(* Logix 5000 AddOnInstructionDefinition export Banner_Q5X_Jam_Param_v4; software revision 33.00; part 2 of 3 *)
(* tags used below, declared in another part *)
   Q5X : Banner_Q5X_Jam_v4;
   Port_Data : Banner_IOL_Port_v4;
   Port : DINT;
   Local_Control : DINT;
   Command_Being_Processed : BOOL;
   Update_Archive : BOOL;
   Index_Write_Inprocess : INT;
   Index_Write_Control : INT;
   Inprocess_Index : DINT;
(* Banner_Q5X_Jam_Param_v4, continued *)

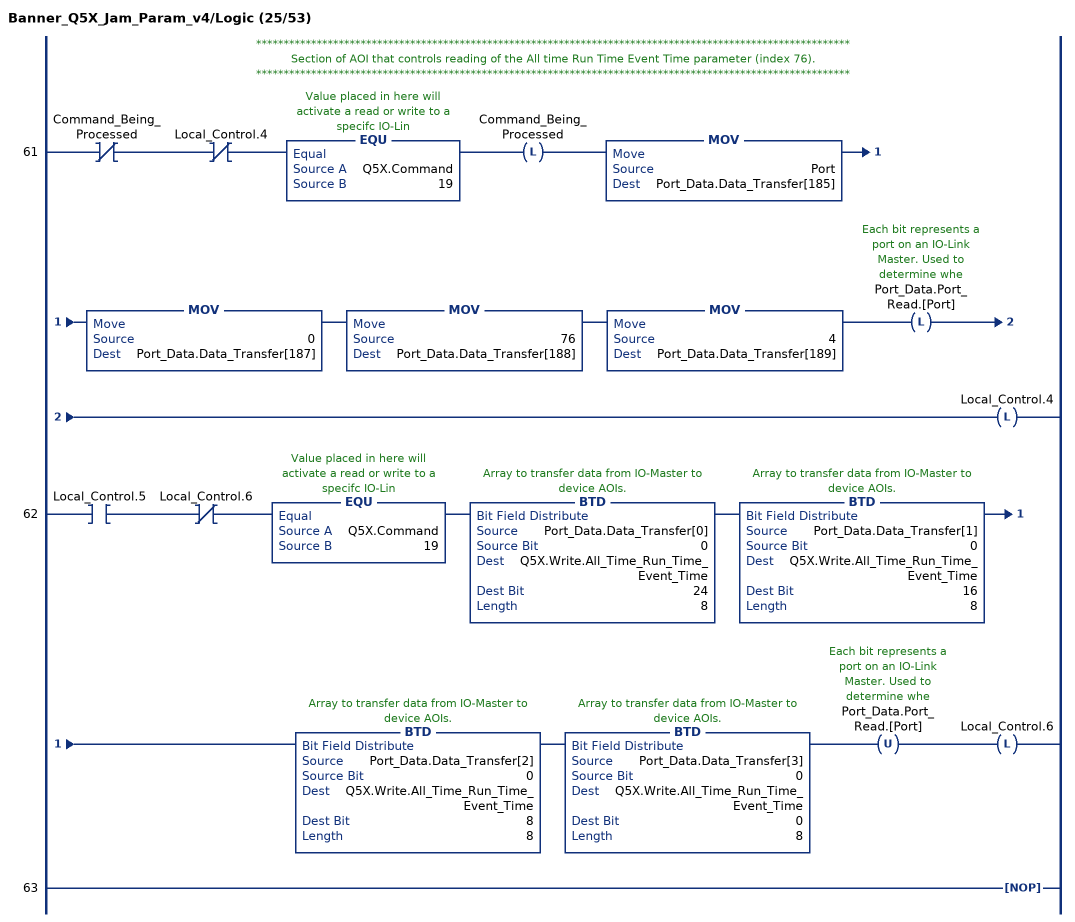
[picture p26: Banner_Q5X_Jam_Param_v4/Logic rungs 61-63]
   // ************************************************************************************************************
   // Section of AOI that controls reading of the All time Run Time Event Time parameter (index 76).
   // ************************************************************************************************************
   61: XIO(Command_Being_Processed)XIO(Local_Control.4)EQU(Q5X.Command,19)OTL(Command_Being_Processed)MOV(Port,Port_Data.Data_Transfer[185])MOV(0,Port_Data.Data_Transfer[187])MOV(76,Port_Data.Data_Transfer[188])MOV(4,Port_Data.Data_Transfer[189])OTL(Port_Data.Port_Read.[Port])OTL(Local_Control.4);
   62: XIC(Local_Control.5)XIO(Local_Control.6)EQU(Q5X.Command,19)BTD(Port_Data.Data_Transfer[0],0,Q5X.Write.All_Time_Run_Time_Event_Time,24,8)BTD(Port_Data.Data_Transfer[1],0,Q5X.Write.All_Time_Run_Time_Event_Time,16,8)BTD(Port_Data.Data_Transfer[2],0,Q5X.Write.All_Time_Run_Time_Event_Time,8,8)BTD(Port_Data.Data_Transfer[3],0,Q5X.Write.All_Time_Run_Time_Event_Time,0,8)OTU(Port_Data.Port_Read.[Port])OTL(Local_Control.6);
   63: NOP();
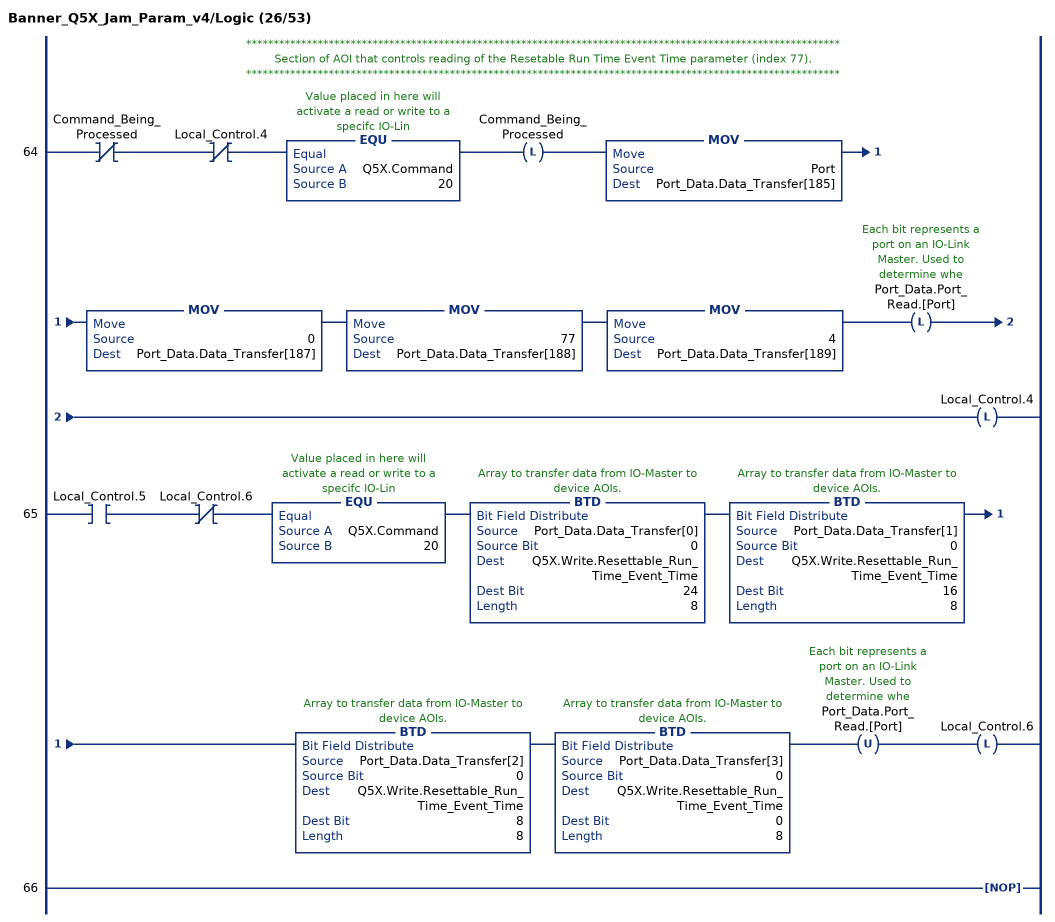
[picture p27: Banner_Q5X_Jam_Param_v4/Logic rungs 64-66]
   // ************************************************************************************************************
   // Section of AOI that controls reading of the Resetable Run Time Event Time parameter (index 77).
   // ************************************************************************************************************
   64: XIO(Command_Being_Processed)XIO(Local_Control.4)EQU(Q5X.Command,20)OTL(Command_Being_Processed)MOV(Port,Port_Data.Data_Transfer[185])MOV(0,Port_Data.Data_Transfer[187])MOV(77,Port_Data.Data_Transfer[188])MOV(4,Port_Data.Data_Transfer[189])OTL(Port_Data.Port_Read.[Port])OTL(Local_Control.4);
   65: XIC(Local_Control.5)XIO(Local_Control.6)EQU(Q5X.Command,20)BTD(Port_Data.Data_Transfer[0],0,Q5X.Write.Resettable_Run_Time_Event_Time,24,8)BTD(Port_Data.Data_Transfer[1],0,Q5X.Write.Resettable_Run_Time_Event_Time,16,8)BTD(Port_Data.Data_Transfer[2],0,Q5X.Write.Resettable_Run_Time_Event_Time,8,8)BTD(Port_Data.Data_Transfer[3],0,Q5X.Write.Resettable_Run_Time_Event_Time,0,8)OTU(Port_Data.Port_Read.[Port])OTL(Local_Control.6);
   66: NOP();
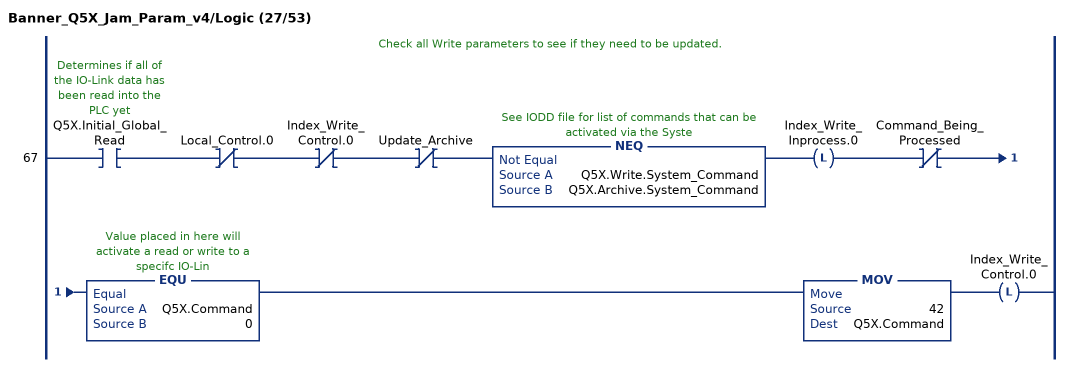
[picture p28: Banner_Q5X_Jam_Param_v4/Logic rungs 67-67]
   // Check all Write parameters to see if they need to be updated.
   67: XIC(Q5X.Initial_Global_Read)XIO(Local_Control.0)XIO(Index_Write_Control.0)XIO(Update_Archive)NEQ(Q5X.Write.System_Command,Q5X.Archive.System_Command)OTL(Index_Write_Inprocess.0)XIO(Command_Being_Processed)EQU(Q5X.Command,0)MOV(42,Q5X.Command)OTL(Index_Write_Control.0);
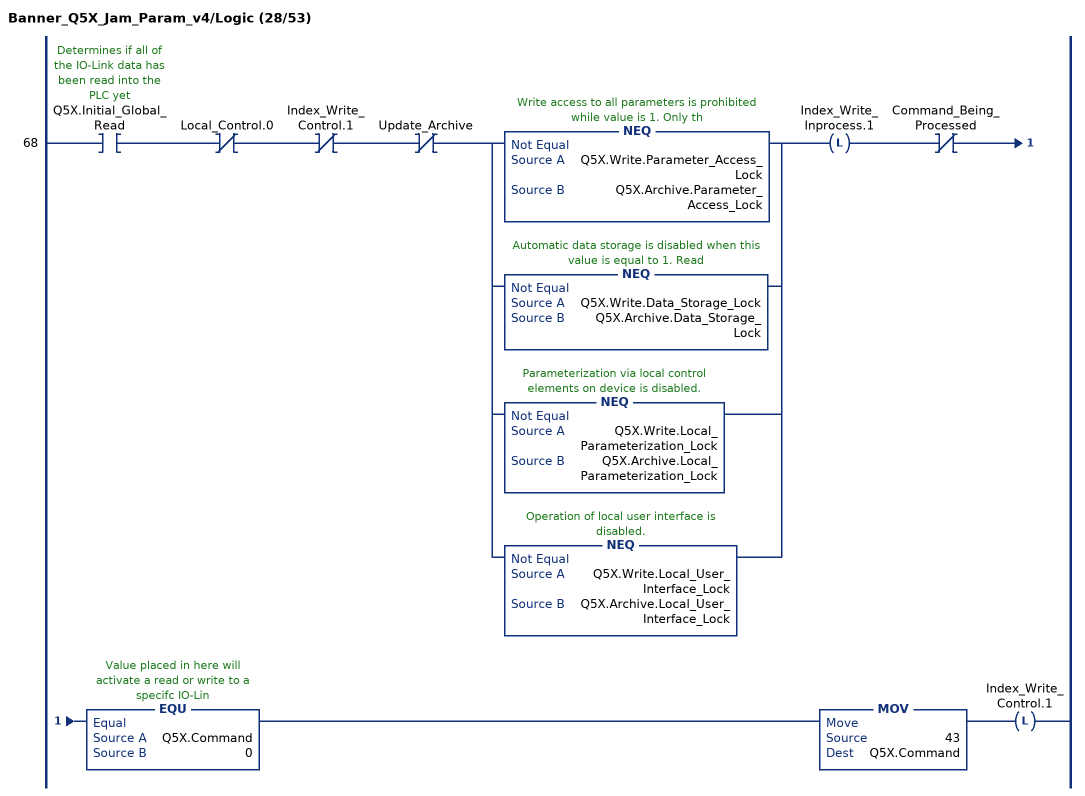
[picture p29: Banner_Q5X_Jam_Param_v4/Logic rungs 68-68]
   68: XIC(Q5X.Initial_Global_Read)XIO(Local_Control.0)XIO(Index_Write_Control.1)XIO(Update_Archive)[NEQ(Q5X.Write.Parameter_Access_Lock,Q5X.Archive.Parameter_Access_Lock) ,NEQ(Q5X.Write.Data_Storage_Lock,Q5X.Archive.Data_Storage_Lock) ,NEQ(Q5X.Write.Local_Parameterization_Lock,Q5X.Archive.Local_Parameterization_Lock) ,NEQ(Q5X.Write.Local_User_Interface_Lock,Q5X.Archive.Local_User_Interface_Lock) ]OTL(Index_Write_Inprocess.1)XIO(Command_Being_Processed)EQU(Q5X.Command,0)MOV(43,Q5X.Command)OTL(Index_Write_Control.1);
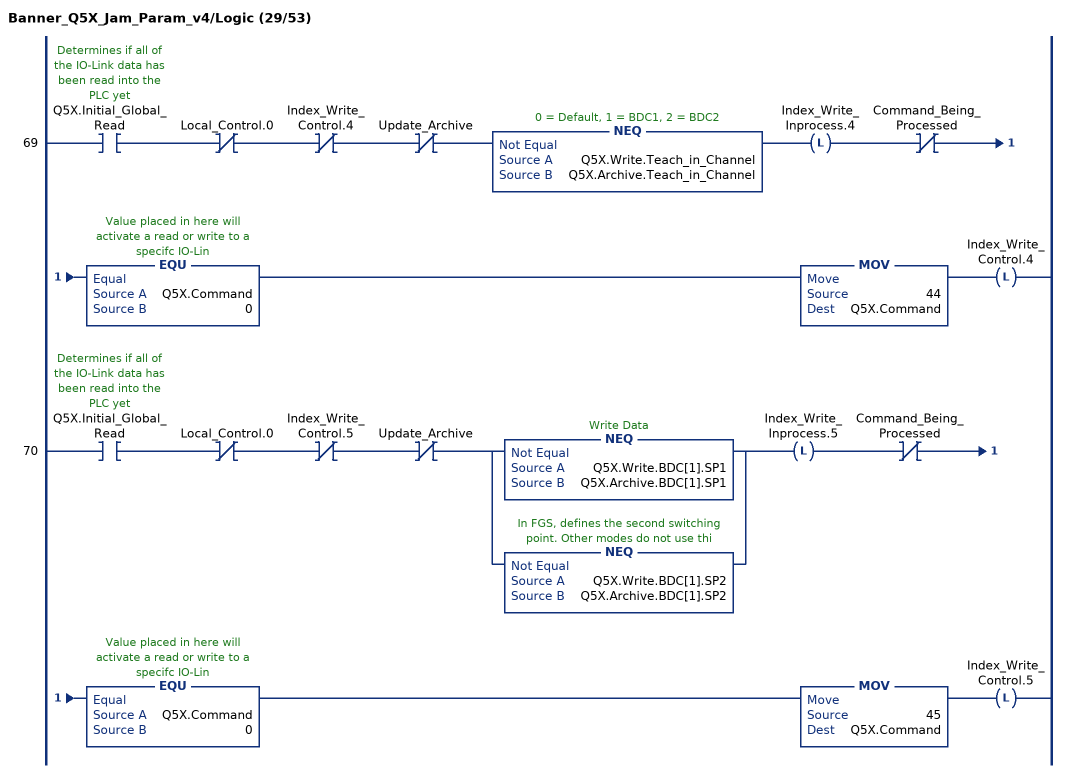
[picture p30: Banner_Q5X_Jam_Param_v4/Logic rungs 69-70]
   69: XIC(Q5X.Initial_Global_Read)XIO(Local_Control.0)XIO(Index_Write_Control.4)XIO(Update_Archive)NEQ(Q5X.Write.Teach_in_Channel,Q5X.Archive.Teach_in_Channel)OTL(Index_Write_Inprocess.4)XIO(Command_Being_Processed)EQU(Q5X.Command,0)MOV(44,Q5X.Command)OTL(Index_Write_Control.4);
   70: XIC(Q5X.Initial_Global_Read)XIO(Local_Control.0)XIO(Index_Write_Control.5)XIO(Update_Archive)[NEQ(Q5X.Write.BDC[1].SP1,Q5X.Archive.BDC[1].SP1) ,NEQ(Q5X.Write.BDC[1].SP2,Q5X.Archive.BDC[1].SP2) ]OTL(Index_Write_Inprocess.5)XIO(Command_Being_Processed)EQU(Q5X.Command,0)MOV(45,Q5X.Command)OTL(Index_Write_Control.5);
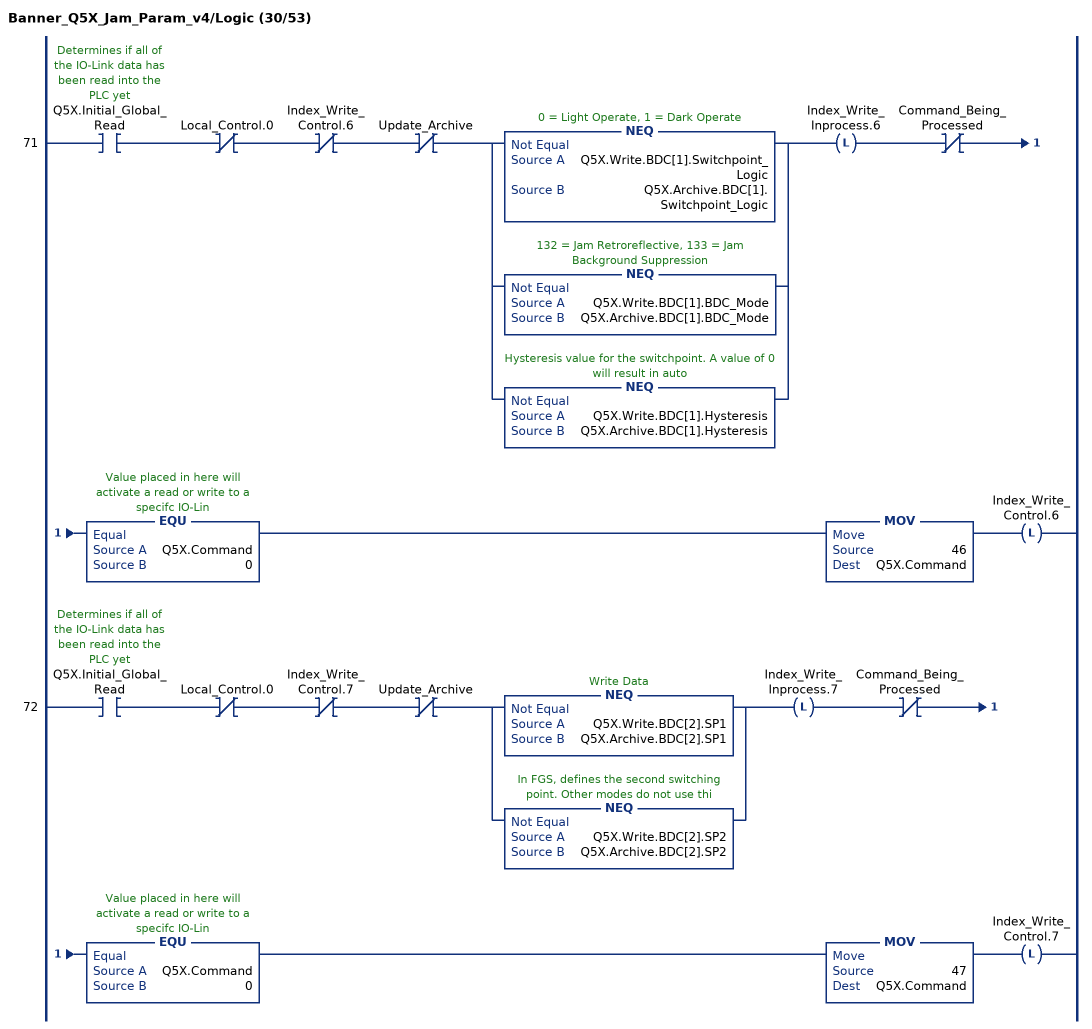
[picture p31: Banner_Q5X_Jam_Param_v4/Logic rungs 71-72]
   71: XIC(Q5X.Initial_Global_Read)XIO(Local_Control.0)XIO(Index_Write_Control.6)XIO(Update_Archive)[NEQ(Q5X.Write.BDC[1].Switchpoint_Logic,Q5X.Archive.BDC[1].Switchpoint_Logic) ,NEQ(Q5X.Write.BDC[1].BDC_Mode,Q5X.Archive.BDC[1].BDC_Mode) ,NEQ(Q5X.Write.BDC[1].Hysteresis,Q5X.Archive.BDC[1].Hysteresis) ]OTL(Index_Write_Inprocess.6)XIO(Command_Being_Processed)EQU(Q5X.Command,0)MOV(46,Q5X.Command)OTL(Index_Write_Control.6);
   72: XIC(Q5X.Initial_Global_Read)XIO(Local_Control.0)XIO(Index_Write_Control.7)XIO(Update_Archive)[NEQ(Q5X.Write.BDC[2].SP1,Q5X.Archive.BDC[2].SP1) ,NEQ(Q5X.Write.BDC[2].SP2,Q5X.Archive.BDC[2].SP2) ]OTL(Index_Write_Inprocess.7)XIO(Command_Being_Processed)EQU(Q5X.Command,0)MOV(47,Q5X.Command)OTL(Index_Write_Control.7);
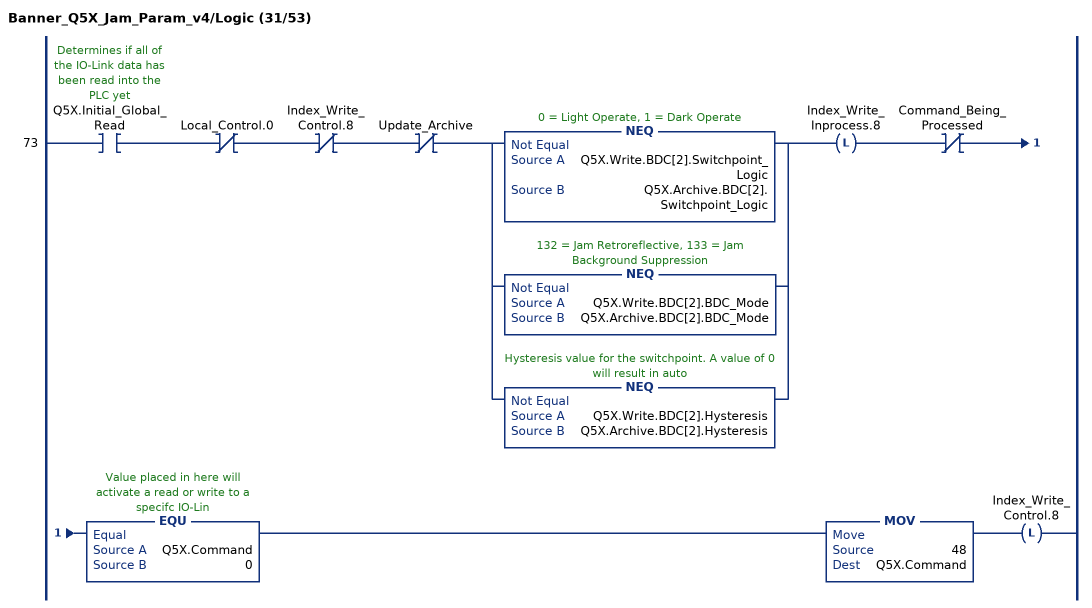
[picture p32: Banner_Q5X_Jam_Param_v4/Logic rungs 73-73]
   73: XIC(Q5X.Initial_Global_Read)XIO(Local_Control.0)XIO(Index_Write_Control.8)XIO(Update_Archive)[NEQ(Q5X.Write.BDC[2].Switchpoint_Logic,Q5X.Archive.BDC[2].Switchpoint_Logic) ,NEQ(Q5X.Write.BDC[2].BDC_Mode,Q5X.Archive.BDC[2].BDC_Mode) ,NEQ(Q5X.Write.BDC[2].Hysteresis,Q5X.Archive.BDC[2].Hysteresis) ]OTL(Index_Write_Inprocess.8)XIO(Command_Being_Processed)EQU(Q5X.Command,0)MOV(48,Q5X.Command)OTL(Index_Write_Control.8);
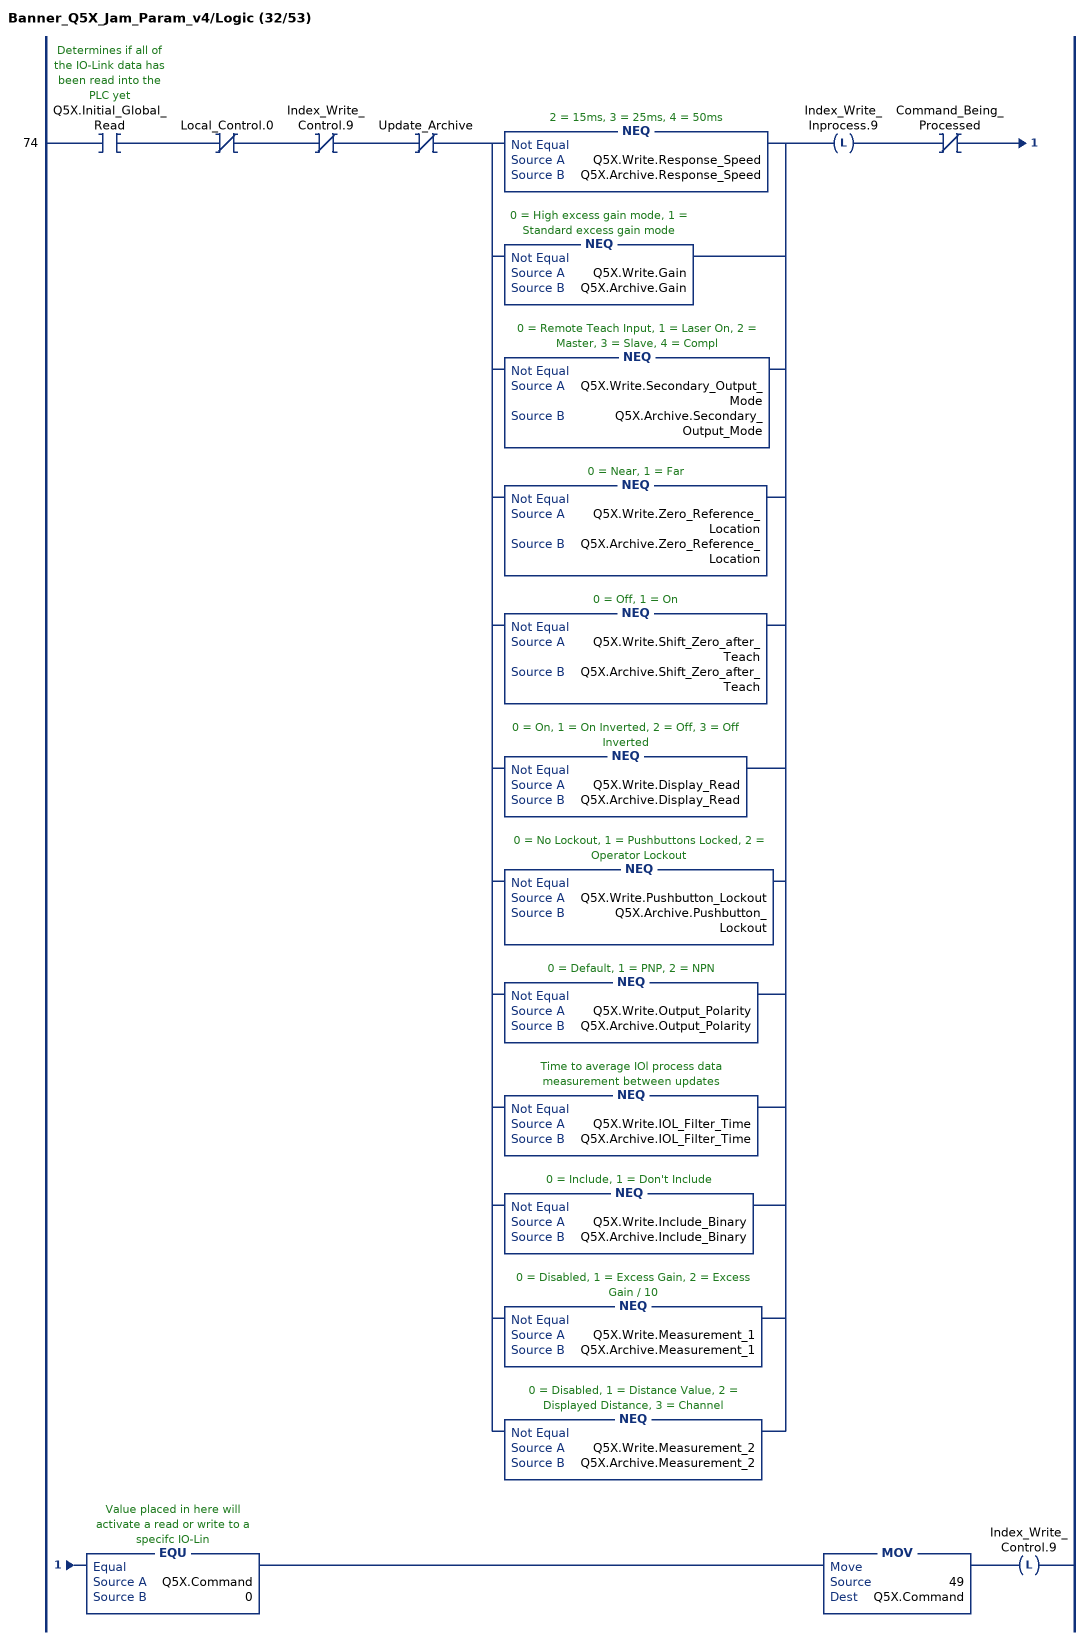
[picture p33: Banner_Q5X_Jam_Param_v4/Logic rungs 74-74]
   74: XIC(Q5X.Initial_Global_Read)XIO(Local_Control.0)XIO(Index_Write_Control.9)XIO(Update_Archive)[NEQ(Q5X.Write.Response_Speed,Q5X.Archive.Response_Speed) ,NEQ(Q5X.Write.Gain,Q5X.Archive.Gain) ,NEQ(Q5X.Write.Secondary_Output_Mode,Q5X.Archive.Secondary_Output_Mode) ,NEQ(Q5X.Write.Zero_Reference_Location,Q5X.Archive.Zero_Reference_Location) ,NEQ(Q5X.Write.Shift_Zero_after_Teach,Q5X.Archive.Shift_Zero_after_Teach) ,NEQ(Q5X.Write.Display_Read,Q5X.Archive.Display_Read) ,NEQ(Q5X.Write.Pushbutton_Lockout,Q5X.Archive.Pushbutton_Lockout) ,NEQ(Q5X.Write.Output_Polarity,Q5X.Archive.Output_Polarity) ,NEQ(Q5X.Write.IOL_Filter_Time,Q5X.Archive.IOL_Filter_Time) ,NEQ(Q5X.Write.Include_Binary,Q5X.Archive.Include_Binary) ,NEQ(Q5X.Write.Measurement_1,Q5X.Archive.Measurement_1) ,NEQ(Q5X.Write.Measurement_2,Q5X.Archive.Measurement_2) ]OTL(Index_Write_Inprocess.9)XIO(Command_Being_Processed)EQU(Q5X.Command,0)MOV(49,Q5X.Command)OTL(Index_Write_Control.9);
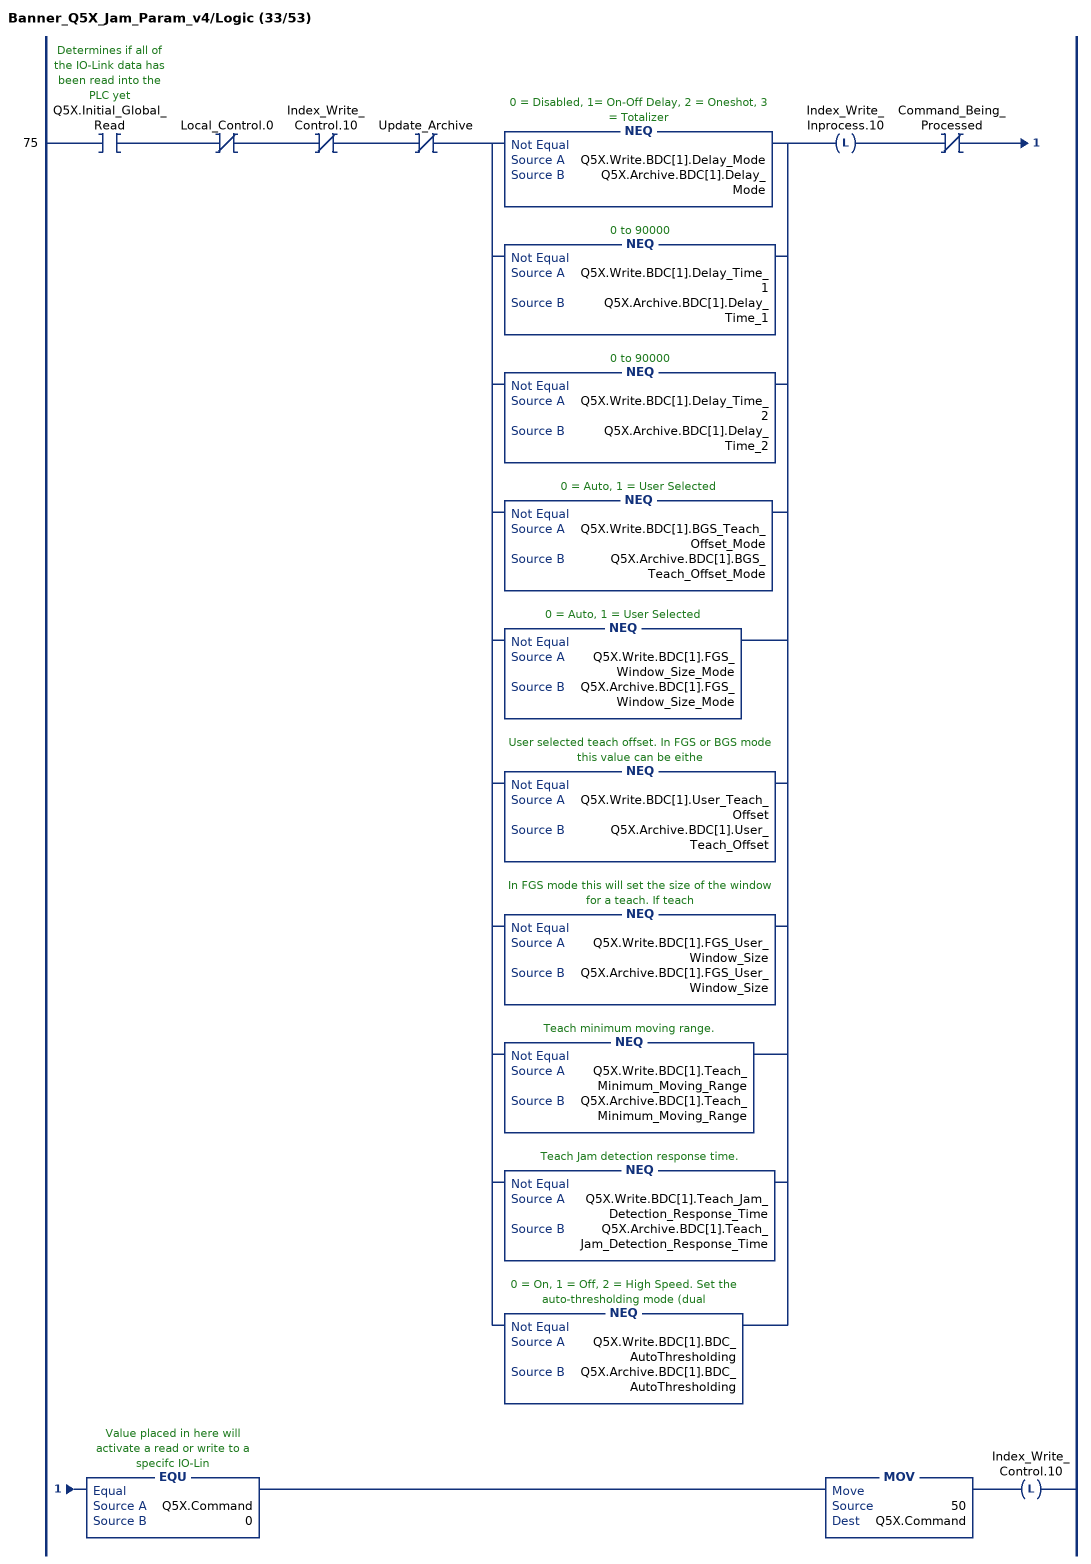
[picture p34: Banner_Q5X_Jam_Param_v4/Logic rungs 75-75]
   75: XIC(Q5X.Initial_Global_Read)XIO(Local_Control.0)XIO(Index_Write_Control.10)XIO(Update_Archive)[NEQ(Q5X.Write.BDC[1].Delay_Mode,Q5X.Archive.BDC[1].Delay_Mode) ,NEQ(Q5X.Write.BDC[1].Delay_Time_1,Q5X.Archive.BDC[1].Delay_Time_1) ,NEQ(Q5X.Write.BDC[1].Delay_Time_2,Q5X.Archive.BDC[1].Delay_Time_2) ,NEQ(Q5X.Write.BDC[1].BGS_Teach_Offset_Mode,Q5X.Archive.BDC[1].BGS_Teach_Offset_Mode) ,NEQ(Q5X.Write.BDC[1].FGS_Window_Size_Mode,Q5X.Archive.BDC[1].FGS_Window_Size_Mode) ,NEQ(Q5X.Write.BDC[1].User_Teach_Offset,Q5X.Archive.BDC[1].User_Teach_Offset) ,NEQ(Q5X.Write.BDC[1].FGS_User_Window_Size,Q5X.Archive.BDC[1].FGS_User_Window_Size) ,NEQ(Q5X.Write.BDC[1].Teach_Minimum_Moving_Range,Q5X.Archive.BDC[1].Teach_Minimum_Moving_Range) ,NEQ(Q5X.Write.BDC[1].Teach_Jam_Detection_Response_Time,Q5X.Archive.BDC[1].Teach_Jam_Detection_Response_Time) ,NEQ(Q5X.Write.BDC[1].BDC_AutoThresholding,Q5X.Archive.BDC[1].BDC_AutoThresholding) ]OTL(Index_Write_Inprocess.10)XIO(Command_Being_Processed)EQU(Q5X.Command,0)MOV(50,Q5X.Command)OTL(Index_Write_Control.10);
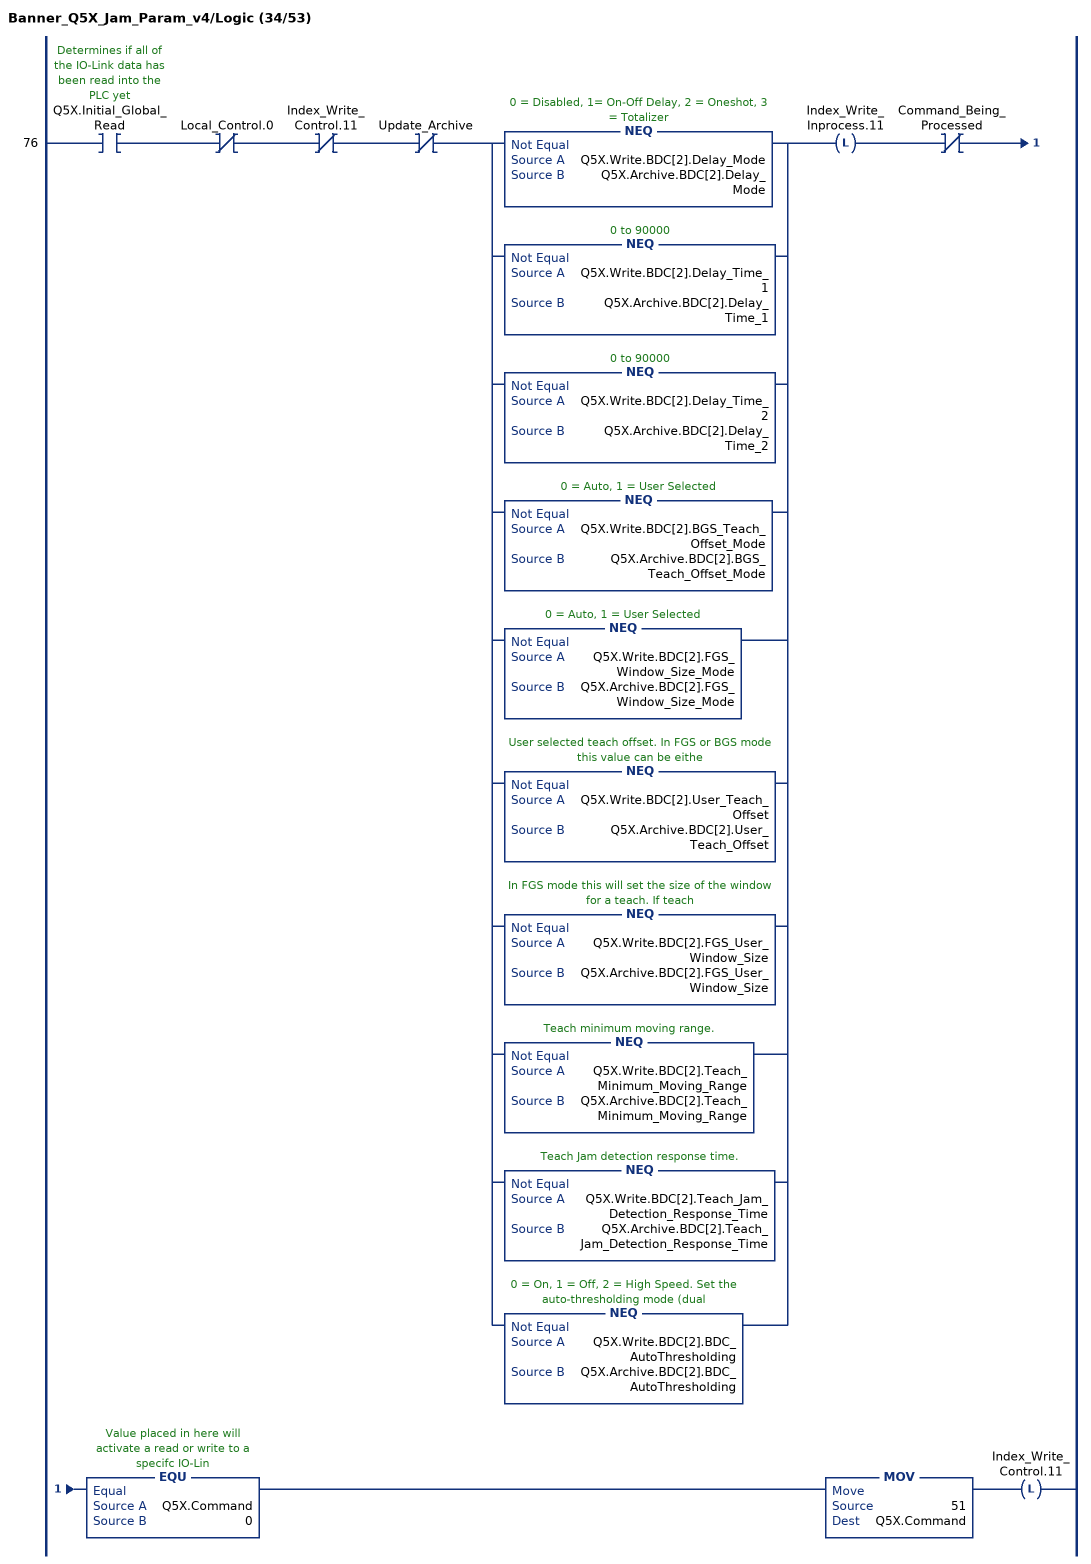
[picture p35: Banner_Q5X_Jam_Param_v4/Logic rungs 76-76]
   76: XIC(Q5X.Initial_Global_Read)XIO(Local_Control.0)XIO(Index_Write_Control.11)XIO(Update_Archive)[NEQ(Q5X.Write.BDC[2].Delay_Mode,Q5X.Archive.BDC[2].Delay_Mode) ,NEQ(Q5X.Write.BDC[2].Delay_Time_1,Q5X.Archive.BDC[2].Delay_Time_1) ,NEQ(Q5X.Write.BDC[2].Delay_Time_2,Q5X.Archive.BDC[2].Delay_Time_2) ,NEQ(Q5X.Write.BDC[2].BGS_Teach_Offset_Mode,Q5X.Archive.BDC[2].BGS_Teach_Offset_Mode) ,NEQ(Q5X.Write.BDC[2].FGS_Window_Size_Mode,Q5X.Archive.BDC[2].FGS_Window_Size_Mode) ,NEQ(Q5X.Write.BDC[2].User_Teach_Offset,Q5X.Archive.BDC[2].User_Teach_Offset) ,NEQ(Q5X.Write.BDC[2].FGS_User_Window_Size,Q5X.Archive.BDC[2].FGS_User_Window_Size) ,NEQ(Q5X.Write.BDC[2].Teach_Minimum_Moving_Range,Q5X.Archive.BDC[2].Teach_Minimum_Moving_Range) ,NEQ(Q5X.Write.BDC[2].Teach_Jam_Detection_Response_Time,Q5X.Archive.BDC[2].Teach_Jam_Detection_Response_Time) ,NEQ(Q5X.Write.BDC[2].BDC_AutoThresholding,Q5X.Archive.BDC[2].BDC_AutoThresholding) ]OTL(Index_Write_Inprocess.11)XIO(Command_Being_Processed)EQU(Q5X.Command,0)MOV(51,Q5X.Command)OTL(Index_Write_Control.11);
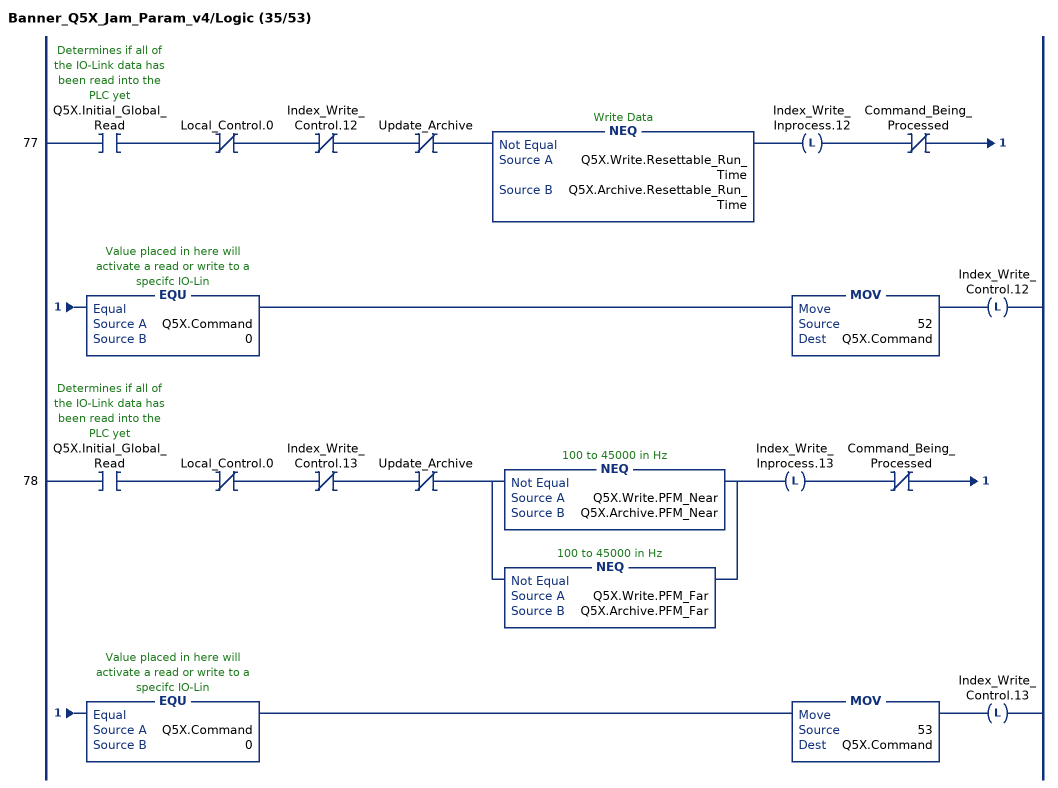
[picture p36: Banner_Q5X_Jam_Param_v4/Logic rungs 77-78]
   77: XIC(Q5X.Initial_Global_Read)XIO(Local_Control.0)XIO(Index_Write_Control.12)XIO(Update_Archive)NEQ(Q5X.Write.Resettable_Run_Time,Q5X.Archive.Resettable_Run_Time)OTL(Index_Write_Inprocess.12)XIO(Command_Being_Processed)EQU(Q5X.Command,0)MOV(52,Q5X.Command)OTL(Index_Write_Control.12);
   78: XIC(Q5X.Initial_Global_Read)XIO(Local_Control.0)XIO(Index_Write_Control.13)XIO(Update_Archive)[NEQ(Q5X.Write.PFM_Near,Q5X.Archive.PFM_Near) ,NEQ(Q5X.Write.PFM_Far,Q5X.Archive.PFM_Far) ]OTL(Index_Write_Inprocess.13)XIO(Command_Being_Processed)EQU(Q5X.Command,0)MOV(53,Q5X.Command)OTL(Index_Write_Control.13);
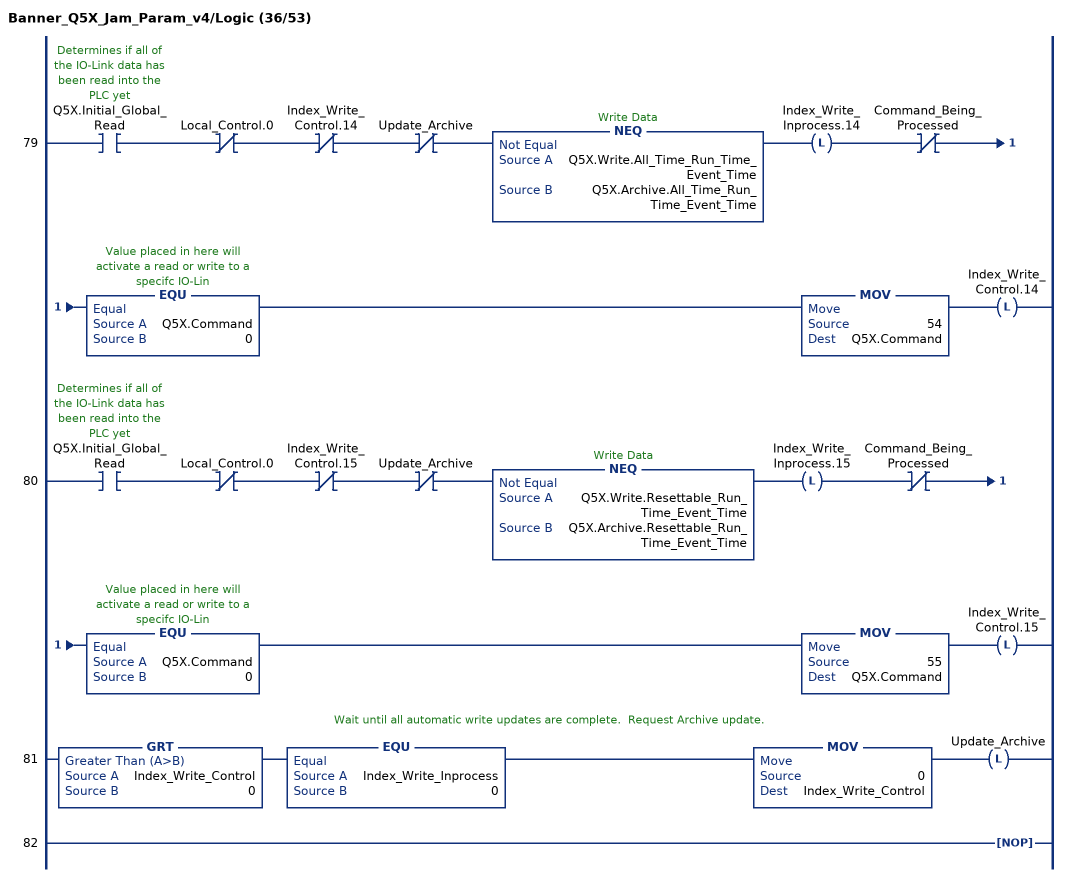
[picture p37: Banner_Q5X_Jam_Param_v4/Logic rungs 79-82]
   79: XIC(Q5X.Initial_Global_Read)XIO(Local_Control.0)XIO(Index_Write_Control.14)XIO(Update_Archive)NEQ(Q5X.Write.All_Time_Run_Time_Event_Time,Q5X.Archive.All_Time_Run_Time_Event_Time)OTL(Index_Write_Inprocess.14)XIO(Command_Being_Processed)EQU(Q5X.Command,0)MOV(54,Q5X.Command)OTL(Index_Write_Control.14);
   80: XIC(Q5X.Initial_Global_Read)XIO(Local_Control.0)XIO(Index_Write_Control.15)XIO(Update_Archive)NEQ(Q5X.Write.Resettable_Run_Time_Event_Time,Q5X.Archive.Resettable_Run_Time_Event_Time)OTL(Index_Write_Inprocess.15)XIO(Command_Being_Processed)EQU(Q5X.Command,0)MOV(55,Q5X.Command)OTL(Index_Write_Control.15);
   // Wait until all automatic write updates are complete.  Request Archive update.
   81: GRT(Index_Write_Control,0)EQU(Index_Write_Inprocess,0)MOV(0,Index_Write_Control)OTL(Update_Archive);
   82: NOP();
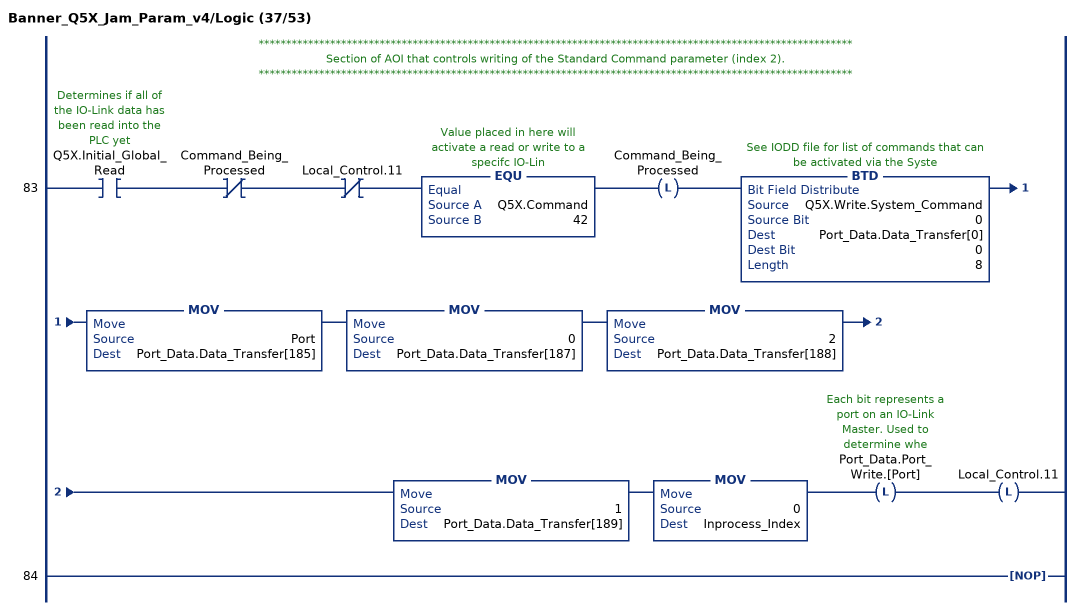
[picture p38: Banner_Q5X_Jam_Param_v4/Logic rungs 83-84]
   // ************************************************************************************************************
   // Section of AOI that controls writing of the Standard Command parameter (index 2).
   // ************************************************************************************************************
   83: XIC(Q5X.Initial_Global_Read)XIO(Command_Being_Processed)XIO(Local_Control.11)EQU(Q5X.Command,42)OTL(Command_Being_Processed)BTD(Q5X.Write.System_Command,0,Port_Data.Data_Transfer[0],0,8)MOV(Port,Port_Data.Data_Transfer[185])MOV(0,Port_Data.Data_Transfer[187])MOV(2,Port_Data.Data_Transfer[188])MOV(1,Port_Data.Data_Transfer[189])MOV(0,Inprocess_Index)OTL(Port_Data.Port_Write.[Port])OTL(Local_Control.11);
   84: NOP();
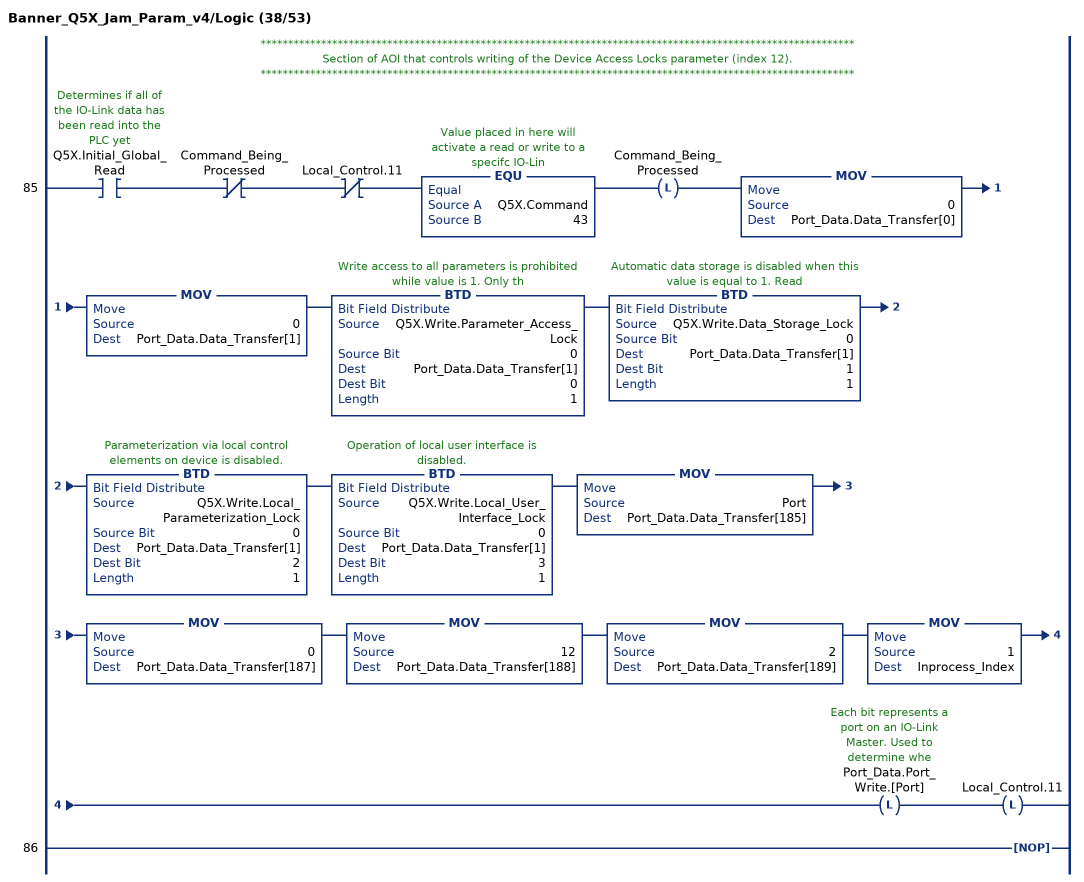
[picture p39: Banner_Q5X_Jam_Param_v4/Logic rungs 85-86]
   // ************************************************************************************************************
   // Section of AOI that controls writing of the Device Access Locks parameter (index 12).
   // ************************************************************************************************************
   85: XIC(Q5X.Initial_Global_Read)XIO(Command_Being_Processed)XIO(Local_Control.11)EQU(Q5X.Command,43)OTL(Command_Being_Processed)MOV(0,Port_Data.Data_Transfer[0])MOV(0,Port_Data.Data_Transfer[1])BTD(Q5X.Write.Parameter_Access_Lock,0,Port_Data.Data_Transfer[1],0,1)BTD(Q5X.Write.Data_Storage_Lock,0,Port_Data.Data_Transfer[1],1,1)BTD(Q5X.Write.Local_Parameterization_Lock,0,Port_Data.Data_Transfer[1],2,1)BTD(Q5X.Write.Local_User_Interface_Lock,0,Port_Data.Data_Transfer[1],3,1)MOV(Port,Port_Data.Data_Transfer[185])MOV(0,Port_Data.Data_Transfer[187])MOV(12,Port_Data.Data_Transfer[188])MOV(2,Port_Data.Data_Transfer[189])MOV(1,Inprocess_Index)OTL(Port_Data.Port_Write.[Port])OTL(Local_Control.11);
   86: NOP();
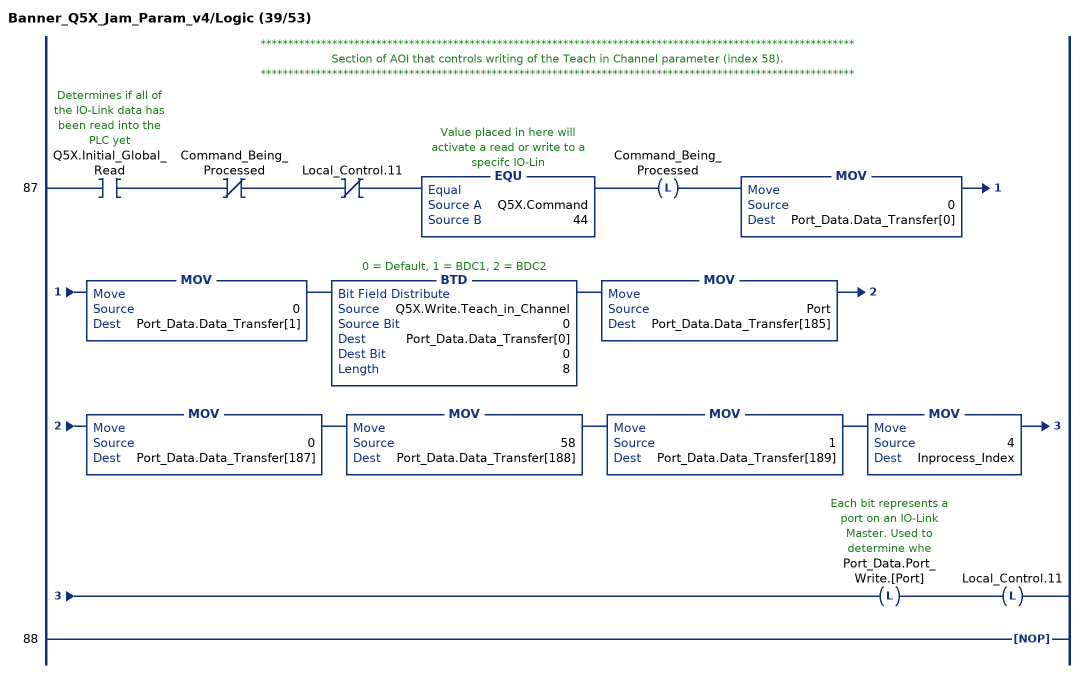
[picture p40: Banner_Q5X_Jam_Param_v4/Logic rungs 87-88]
   // ************************************************************************************************************
   // Section of AOI that controls writing of the Teach in Channel parameter (index 58).
   // ************************************************************************************************************
   87: XIC(Q5X.Initial_Global_Read)XIO(Command_Being_Processed)XIO(Local_Control.11)EQU(Q5X.Command,44)OTL(Command_Being_Processed)MOV(0,Port_Data.Data_Transfer[0])MOV(0,Port_Data.Data_Transfer[1])BTD(Q5X.Write.Teach_in_Channel,0,Port_Data.Data_Transfer[0],0,8)MOV(Port,Port_Data.Data_Transfer[185])MOV(0,Port_Data.Data_Transfer[187])MOV(58,Port_Data.Data_Transfer[188])MOV(1,Port_Data.Data_Transfer[189])MOV(4,Inprocess_Index)OTL(Port_Data.Port_Write.[Port])OTL(Local_Control.11);
   88: NOP();
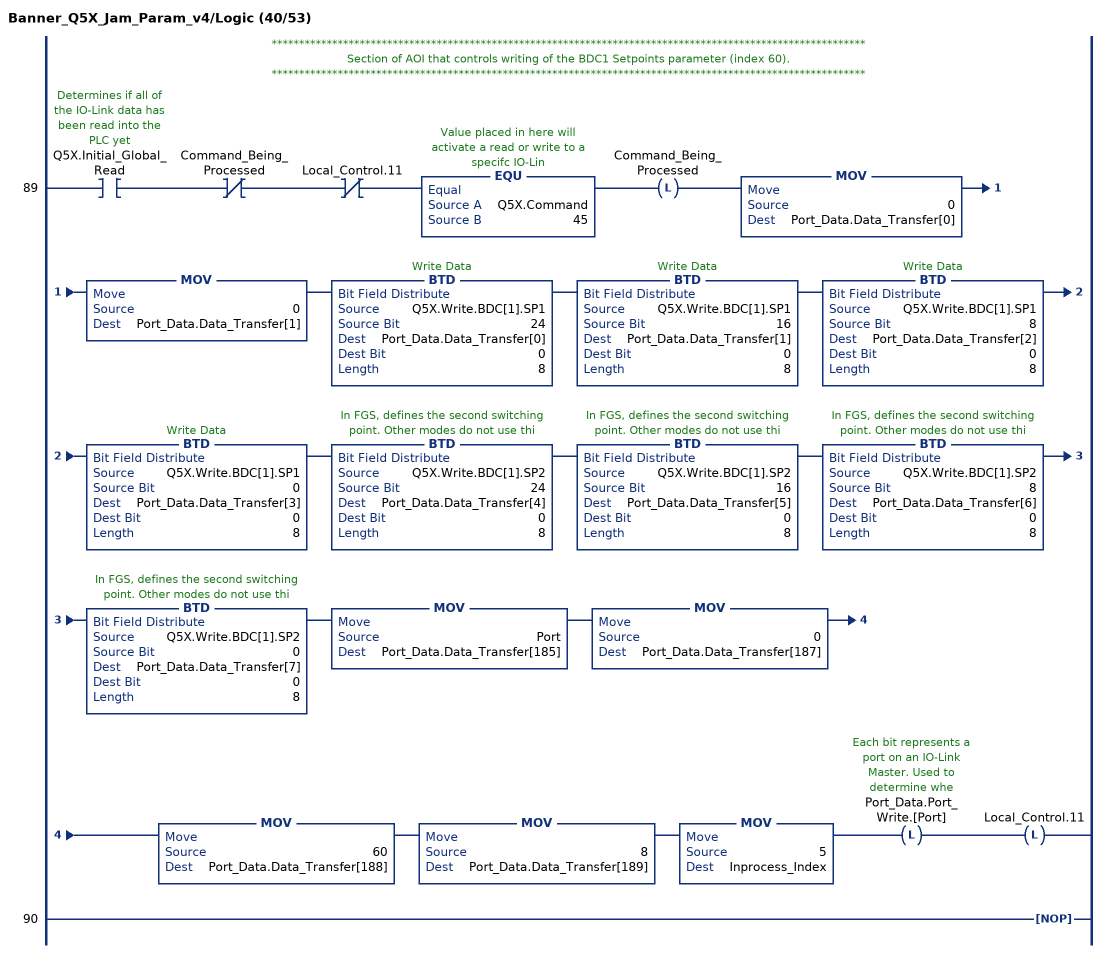
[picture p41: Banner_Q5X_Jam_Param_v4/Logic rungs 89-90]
   // ************************************************************************************************************
   // Section of AOI that controls writing of the BDC1 Setpoints parameter (index 60).
   // ************************************************************************************************************
   89: XIC(Q5X.Initial_Global_Read)XIO(Command_Being_Processed)XIO(Local_Control.11)EQU(Q5X.Command,45)OTL(Command_Being_Processed)MOV(0,Port_Data.Data_Transfer[0])MOV(0,Port_Data.Data_Transfer[1])BTD(Q5X.Write.BDC[1].SP1,24,Port_Data.Data_Transfer[0],0,8)BTD(Q5X.Write.BDC[1].SP1,16,Port_Data.Data_Transfer[1],0,8)BTD(Q5X.Write.BDC[1].SP1,8,Port_Data.Data_Transfer[2],0,8)BTD(Q5X.Write.BDC[1].SP1,0,Port_Data.Data_Transfer[3],0,8)BTD(Q5X.Write.BDC[1].SP2,24,Port_Data.Data_Transfer[4],0,8)BTD(Q5X.Write.BDC[1].SP2,16,Port_Data.Data_Transfer[5],0,8)BTD(Q5X.Write.BDC[1].SP2,8,Port_Data.Data_Transfer[6],0,8)BTD(Q5X.Write.BDC[1].SP2,0,Port_Data.Data_Transfer[7],0,8)MOV(Port,Port_Data.Data_Transfer[185])MOV(0,Port_Data.Data_Transfer[187])MOV(60,Port_Data.Data_Transfer[188])MOV(8,Port_Data.Data_Transfer[189])MOV(5,Inprocess_Index)OTL(Port_Data.Port_Write.[Port])OTL(Local_Control.11);
   90: NOP();
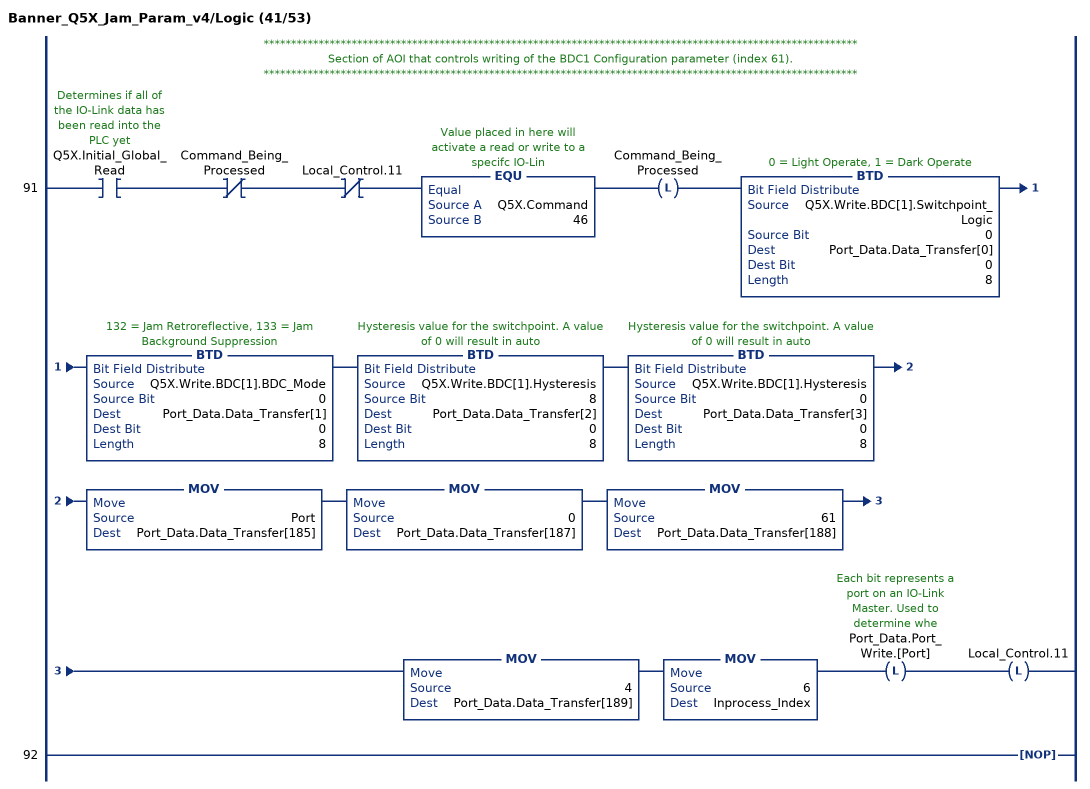
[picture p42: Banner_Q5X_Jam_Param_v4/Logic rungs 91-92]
   // ************************************************************************************************************
   // Section of AOI that controls writing of the BDC1 Configuration parameter (index 61).
   // ************************************************************************************************************
   91: XIC(Q5X.Initial_Global_Read)XIO(Command_Being_Processed)XIO(Local_Control.11)EQU(Q5X.Command,46)OTL(Command_Being_Processed)BTD(Q5X.Write.BDC[1].Switchpoint_Logic,0,Port_Data.Data_Transfer[0],0,8)BTD(Q5X.Write.BDC[1].BDC_Mode,0,Port_Data.Data_Transfer[1],0,8)BTD(Q5X.Write.BDC[1].Hysteresis,8,Port_Data.Data_Transfer[2],0,8)BTD(Q5X.Write.BDC[1].Hysteresis,0,Port_Data.Data_Transfer[3],0,8)MOV(Port,Port_Data.Data_Transfer[185])MOV(0,Port_Data.Data_Transfer[187])MOV(61,Port_Data.Data_Transfer[188])MOV(4,Port_Data.Data_Transfer[189])MOV(6,Inprocess_Index)OTL(Port_Data.Port_Write.[Port])OTL(Local_Control.11);
   92: NOP();
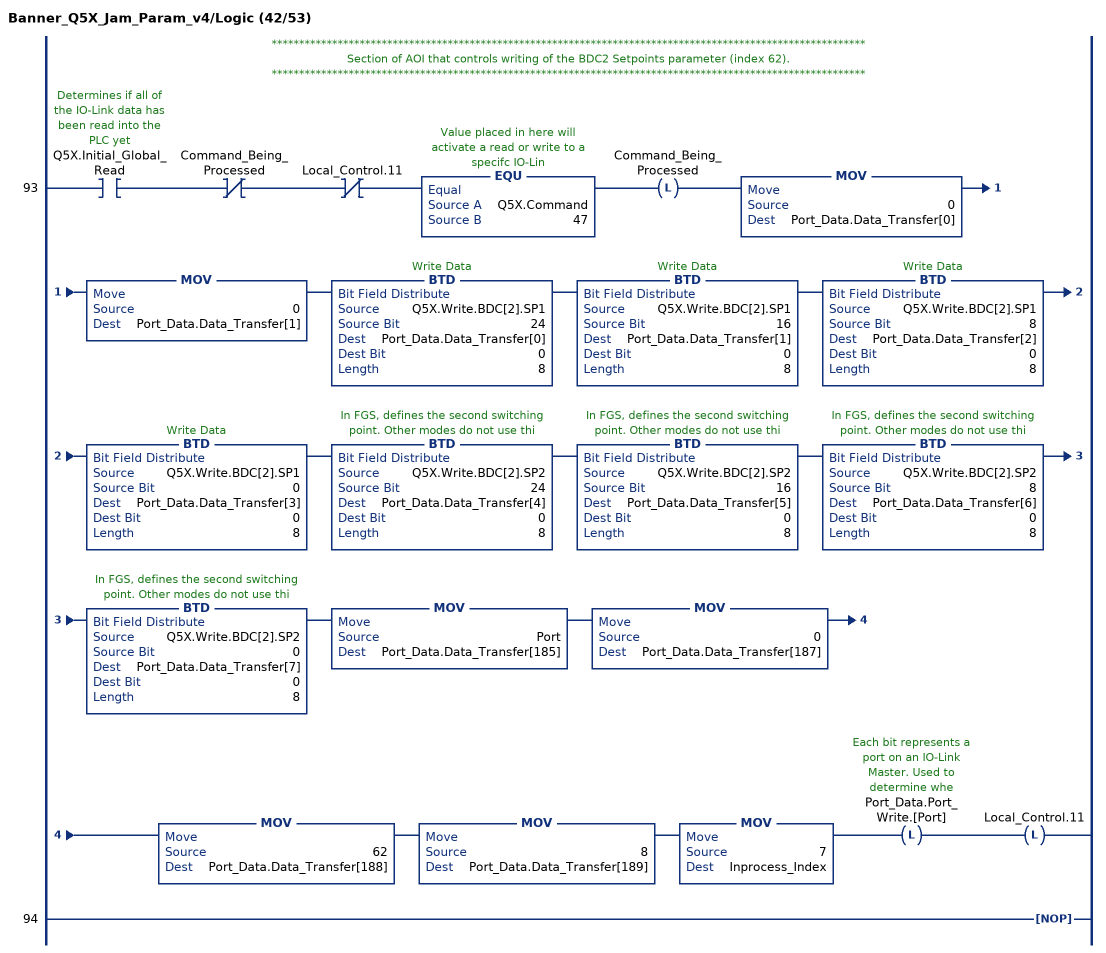
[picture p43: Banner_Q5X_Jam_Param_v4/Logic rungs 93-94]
   // ************************************************************************************************************
   // Section of AOI that controls writing of the BDC2 Setpoints parameter (index 62).
   // ************************************************************************************************************
   93: XIC(Q5X.Initial_Global_Read)XIO(Command_Being_Processed)XIO(Local_Control.11)EQU(Q5X.Command,47)OTL(Command_Being_Processed)MOV(0,Port_Data.Data_Transfer[0])MOV(0,Port_Data.Data_Transfer[1])BTD(Q5X.Write.BDC[2].SP1,24,Port_Data.Data_Transfer[0],0,8)BTD(Q5X.Write.BDC[2].SP1,16,Port_Data.Data_Transfer[1],0,8)BTD(Q5X.Write.BDC[2].SP1,8,Port_Data.Data_Transfer[2],0,8)BTD(Q5X.Write.BDC[2].SP1,0,Port_Data.Data_Transfer[3],0,8)BTD(Q5X.Write.BDC[2].SP2,24,Port_Data.Data_Transfer[4],0,8)BTD(Q5X.Write.BDC[2].SP2,16,Port_Data.Data_Transfer[5],0,8)BTD(Q5X.Write.BDC[2].SP2,8,Port_Data.Data_Transfer[6],0,8)BTD(Q5X.Write.BDC[2].SP2,0,Port_Data.Data_Transfer[7],0,8)MOV(Port,Port_Data.Data_Transfer[185])MOV(0,Port_Data.Data_Transfer[187])MOV(62,Port_Data.Data_Transfer[188])MOV(8,Port_Data.Data_Transfer[189])MOV(7,Inprocess_Index)OTL(Port_Data.Port_Write.[Port])OTL(Local_Control.11);
   94: NOP();
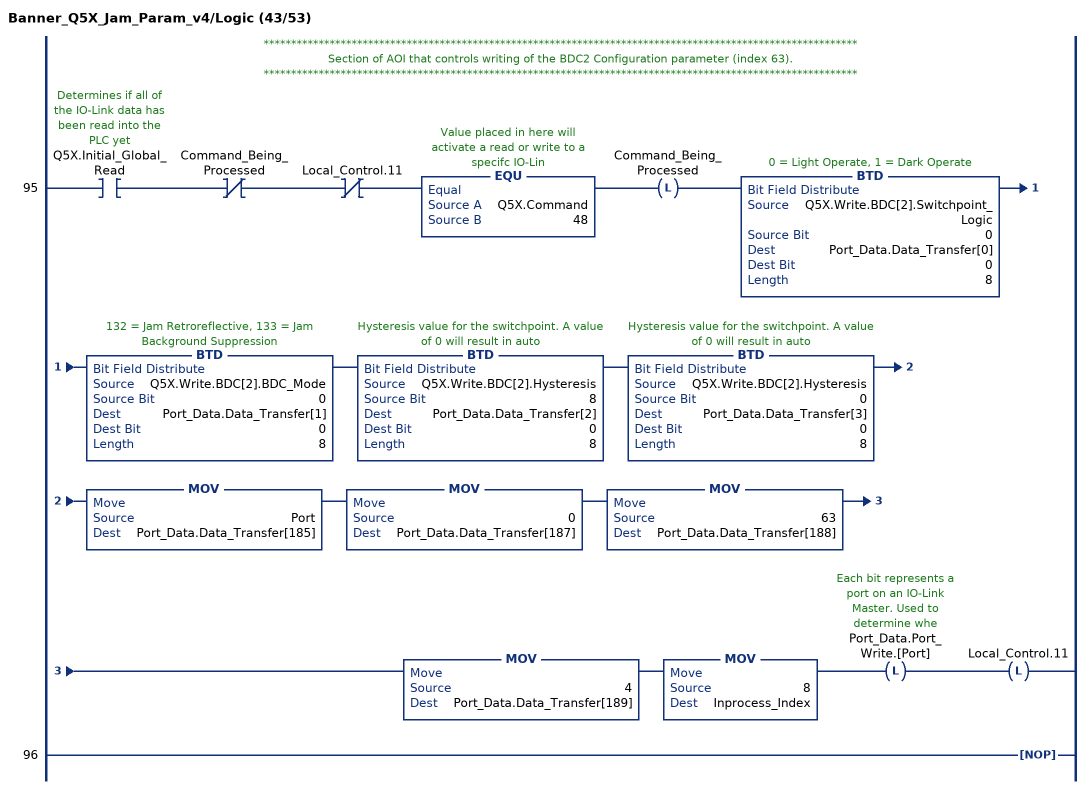
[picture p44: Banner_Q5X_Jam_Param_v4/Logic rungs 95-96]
   // ************************************************************************************************************
   // Section of AOI that controls writing of the BDC2 Configuration parameter (index 63).
   // ************************************************************************************************************
   95: XIC(Q5X.Initial_Global_Read)XIO(Command_Being_Processed)XIO(Local_Control.11)EQU(Q5X.Command,48)OTL(Command_Being_Processed)BTD(Q5X.Write.BDC[2].Switchpoint_Logic,0,Port_Data.Data_Transfer[0],0,8)BTD(Q5X.Write.BDC[2].BDC_Mode,0,Port_Data.Data_Transfer[1],0,8)BTD(Q5X.Write.BDC[2].Hysteresis,8,Port_Data.Data_Transfer[2],0,8)BTD(Q5X.Write.BDC[2].Hysteresis,0,Port_Data.Data_Transfer[3],0,8)MOV(Port,Port_Data.Data_Transfer[185])MOV(0,Port_Data.Data_Transfer[187])MOV(63,Port_Data.Data_Transfer[188])MOV(4,Port_Data.Data_Transfer[189])MOV(8,Inprocess_Index)OTL(Port_Data.Port_Write.[Port])OTL(Local_Control.11);
   96: NOP();
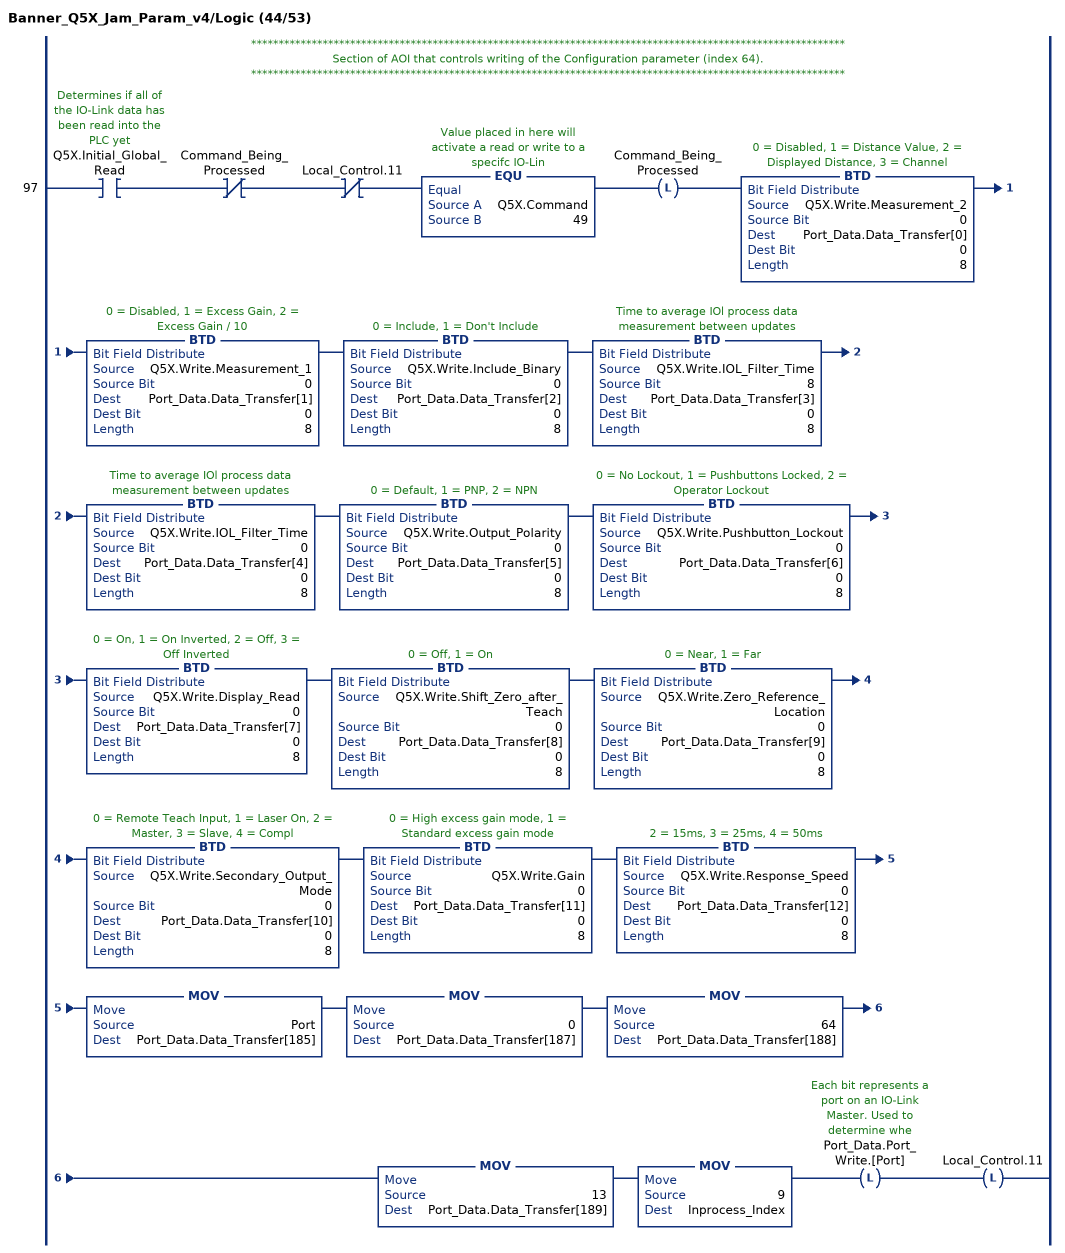
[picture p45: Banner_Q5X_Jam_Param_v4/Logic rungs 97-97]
   // ************************************************************************************************************
   // Section of AOI that controls writing of the Configuration parameter (index 64).
   // ************************************************************************************************************
   97: XIC(Q5X.Initial_Global_Read)XIO(Command_Being_Processed)XIO(Local_Control.11)EQU(Q5X.Command,49)OTL(Command_Being_Processed)BTD(Q5X.Write.Measurement_2,0,Port_Data.Data_Transfer[0],0,8)BTD(Q5X.Write.Measurement_1,0,Port_Data.Data_Transfer[1],0,8)BTD(Q5X.Write.Include_Binary,0,Port_Data.Data_Transfer[2],0,8)BTD(Q5X.Write.IOL_Filter_Time,8,Port_Data.Data_Transfer[3],0,8)BTD(Q5X.Write.IOL_Filter_Time,0,Port_Data.Data_Transfer[4],0,8)BTD(Q5X.Write.Output_Polarity,0,Port_Data.Data_Transfer[5],0,8)BTD(Q5X.Write.Pushbutton_Lockout,0,Port_Data.Data_Transfer[6],0,8)BTD(Q5X.Write.Display_Read,0,Port_Data.Data_Transfer[7],0,8)BTD(Q5X.Write.Shift_Zero_after_Teach,0,Port_Data.Data_Transfer[8],0,8)BTD(Q5X.Write.Zero_Reference_Location,0,Port_Data.Data_Transfer[9],0,8)BTD(Q5X.Write.Secondary_Output_Mode,0,Port_Data.Data_Transfer[10],0,8)BTD(Q5X.Write.Gain,0,Port_Data.Data_Transfer[11],0,8)BTD(Q5X.Write.Response_Speed,0,Port_Data.Data_Transfer[12],0,8)MOV(Port,Port_Data.Data_Transfer[185])MOV(0,Port_Data.Data_Transfer[187])MOV(64,Port_Data.Data_Transfer[188])MOV(13,Port_Data.Data_Transfer[189])MOV(9,Inprocess_Index)OTL(Port_Data.Port_Write.[Port])OTL(Local_Control.11);
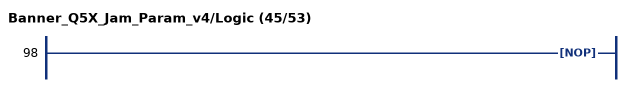
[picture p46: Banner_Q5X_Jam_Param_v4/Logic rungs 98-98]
   98: NOP();
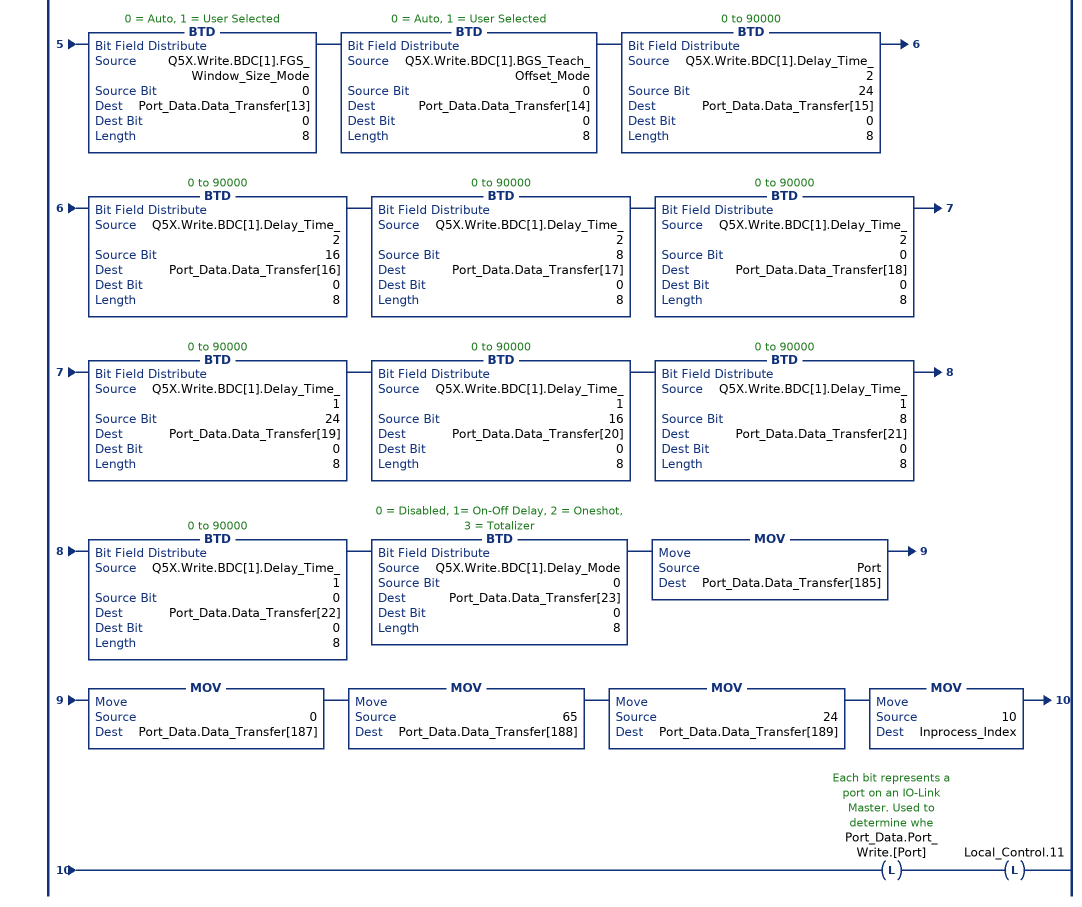
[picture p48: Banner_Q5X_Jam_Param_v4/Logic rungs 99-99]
   // ************************************************************************************************************
   // Section of AOI that controls writing of the BDC1 Vendor Specific Configuration parameter (index 65).
   // ************************************************************************************************************
   99: XIC(Q5X.Initial_Global_Read)XIO(Command_Being_Processed)XIO(Local_Control.11)EQU(Q5X.Command,50)OTL(Command_Being_Processed)BTD(Q5X.Write.BDC[1].BDC_AutoThresholding,0,Port_Data.Data_Transfer[0],0,8)BTD(Q5X.Write.BDC[1].Teach_Jam_Detection_Response_Time,24,Port_Data.Data_Transfer[1],0,8)BTD(Q5X.Write.BDC[1].Teach_Jam_Detection_Response_Time,16,Port_Data.Data_Transfer[2],0,8)BTD(Q5X.Write.BDC[1].Teach_Jam_Detection_Response_Time,8,Port_Data.Data_Transfer[3],0,8)BTD(Q5X.Write.BDC[1].Teach_Jam_Detection_Response_Time,0,Port_Data.Data_Transfer[4],0,8)BTD(Q5X.Write.BDC[1].Teach_Minimum_Moving_Range,24,Port_Data.Data_Transfer[5],0,8)BTD(Q5X.Write.BDC[1].Teach_Minimum_Moving_Range,16,Port_Data.Data_Transfer[6],0,8)BTD(Q5X.Write.BDC[1].Teach_Minimum_Moving_Range,8,Port_Data.Data_Transfer[7],0,8)BTD(Q5X.Write.BDC[1].Teach_Minimum_Moving_Range,0,Port_Data.Data_Transfer[8],0,8)BTD(Q5X.Write.BDC[1].FGS_User_Window_Size,8,Port_Data.Data_Transfer[9],0,8)BTD(Q5X.Write.BDC[1].FGS_User_Window_Size,0,Port_Data.Data_Transfer[10],0,8)BTD(Q5X.Write.BDC[1].User_Teach_Offset,8,Port_Data.Data_Transfer[11],0,8)BTD(Q5X.Write.BDC[1].User_Teach_Offset,0,Port_Data.Data_Transfer[12],0,8)BTD(Q5X.Write.BDC[1].FGS_Window_Size_Mode,0,Port_Data.Data_Transfer[13],0,8)BTD(Q5X.Write.BDC[1].BGS_Teach_Offset_Mode,0,Port_Data.Data_Transfer[14],0,8)BTD(Q5X.Write.BDC[1].Delay_Time_2,24,Port_Data.Data_Transfer[15],0,8)BTD(Q5X.Write.BDC[1].Delay_Time_2,16,Port_Data.Data_Transfer[16],0,8)BTD(Q5X.Write.BDC[1].Delay_Time_2,8,Port_Data.Data_Transfer[17],0,8)BTD(Q5X.Write.BDC[1].Delay_Time_2,0,Port_Data.Data_Transfer[18],0,8)BTD(Q5X.Write.BDC[1].Delay_Time_1,24,Port_Data.Data_Transfer[19],0,8)BTD(Q5X.Write.BDC[1].Delay_Time_1,16,Port_Data.Data_Transfer[20],0,8)BTD(Q5X.Write.BDC[1].Delay_Time_1,8,Port_Data.Data_Transfer[21],0,8)BTD(Q5X.Write.BDC[1].Delay_Time_1,0,Port_Data.Data_Transfer[22],0,8)BTD(Q5X.Write.BDC[1].Delay_Mode,0,Port_Data.Data_Transfer[23],0,8)MOV(Port,Port_Data.Data_Transfer[185])MOV(0,Port_Data.Data_Transfer[187])MOV(65,Port_Data.Data_Transfer[188])MOV(24,Port_Data.Data_Transfer[189])MOV(10,Inprocess_Index)OTL(Port_Data.Port_Write.[Port])OTL(Local_Control.11);
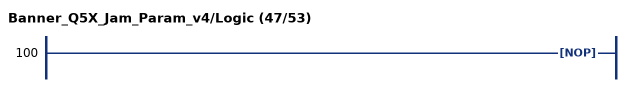
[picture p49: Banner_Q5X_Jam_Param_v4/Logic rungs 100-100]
   100: NOP();
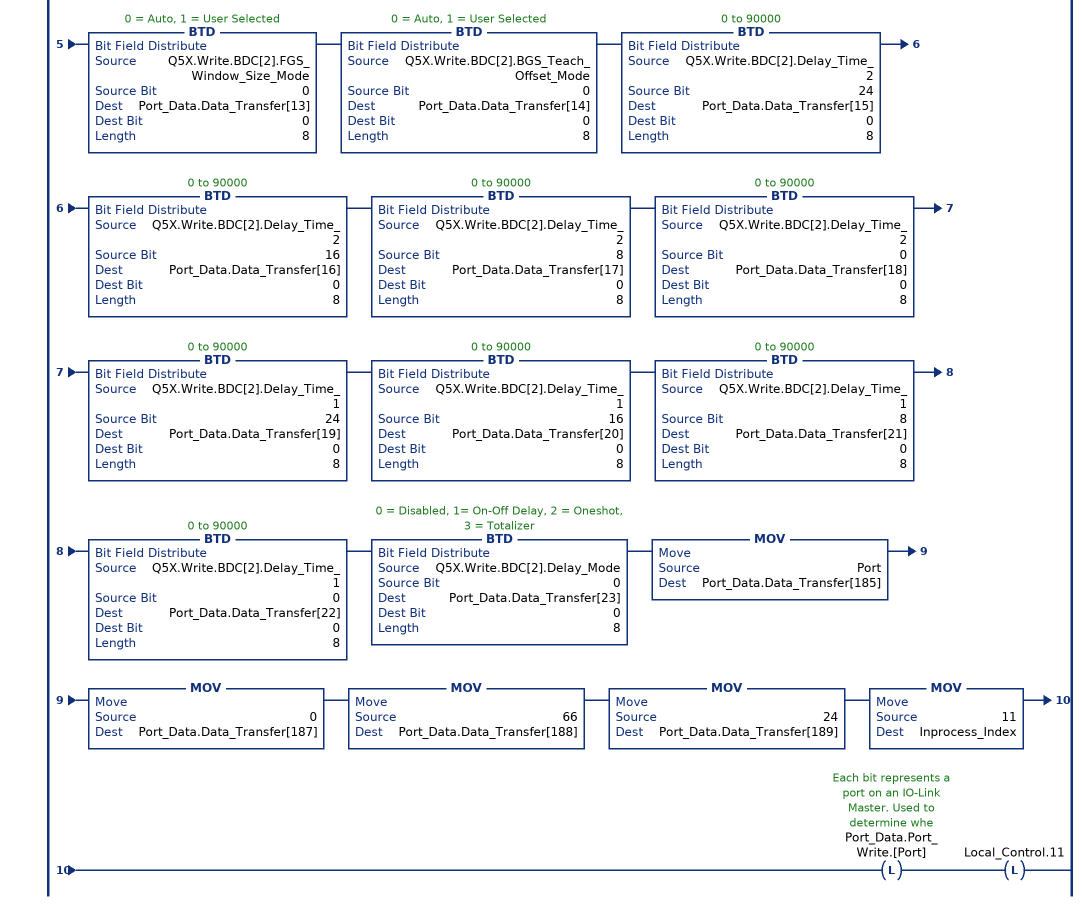
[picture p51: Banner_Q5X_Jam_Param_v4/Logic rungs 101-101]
   // ************************************************************************************************************
   // Section of AOI that controls writing of the BDC2 Vendor Specific Configuration parameter (index 66).
   // ************************************************************************************************************
   101: XIC(Q5X.Initial_Global_Read)XIO(Command_Being_Processed)XIO(Local_Control.11)EQU(Q5X.Command,51)OTL(Command_Being_Processed)BTD(Q5X.Write.BDC[2].BDC_AutoThresholding,0,Port_Data.Data_Transfer[0],0,8)BTD(Q5X.Write.BDC[2].Teach_Jam_Detection_Response_Time,24,Port_Data.Data_Transfer[1],0,8)BTD(Q5X.Write.BDC[2].Teach_Jam_Detection_Response_Time,16,Port_Data.Data_Transfer[2],0,8)BTD(Q5X.Write.BDC[2].Teach_Jam_Detection_Response_Time,8,Port_Data.Data_Transfer[3],0,8)BTD(Q5X.Write.BDC[2].Teach_Jam_Detection_Response_Time,0,Port_Data.Data_Transfer[4],0,8)BTD(Q5X.Write.BDC[2].Teach_Minimum_Moving_Range,24,Port_Data.Data_Transfer[5],0,8)BTD(Q5X.Write.BDC[2].Teach_Minimum_Moving_Range,16,Port_Data.Data_Transfer[6],0,8)BTD(Q5X.Write.BDC[2].Teach_Minimum_Moving_Range,8,Port_Data.Data_Transfer[7],0,8)BTD(Q5X.Write.BDC[2].Teach_Minimum_Moving_Range,0,Port_Data.Data_Transfer[8],0,8)BTD(Q5X.Write.BDC[2].FGS_User_Window_Size,8,Port_Data.Data_Transfer[9],0,8)BTD(Q5X.Write.BDC[2].FGS_User_Window_Size,0,Port_Data.Data_Transfer[10],0,8)BTD(Q5X.Write.BDC[2].User_Teach_Offset,8,Port_Data.Data_Transfer[11],0,8)BTD(Q5X.Write.BDC[2].User_Teach_Offset,0,Port_Data.Data_Transfer[12],0,8)BTD(Q5X.Write.BDC[2].FGS_Window_Size_Mode,0,Port_Data.Data_Transfer[13],0,8)BTD(Q5X.Write.BDC[2].BGS_Teach_Offset_Mode,0,Port_Data.Data_Transfer[14],0,8)BTD(Q5X.Write.BDC[2].Delay_Time_2,24,Port_Data.Data_Transfer[15],0,8)BTD(Q5X.Write.BDC[2].Delay_Time_2,16,Port_Data.Data_Transfer[16],0,8)BTD(Q5X.Write.BDC[2].Delay_Time_2,8,Port_Data.Data_Transfer[17],0,8)BTD(Q5X.Write.BDC[2].Delay_Time_2,0,Port_Data.Data_Transfer[18],0,8)BTD(Q5X.Write.BDC[2].Delay_Time_1,24,Port_Data.Data_Transfer[19],0,8)BTD(Q5X.Write.BDC[2].Delay_Time_1,16,Port_Data.Data_Transfer[20],0,8)BTD(Q5X.Write.BDC[2].Delay_Time_1,8,Port_Data.Data_Transfer[21],0,8)BTD(Q5X.Write.BDC[2].Delay_Time_1,0,Port_Data.Data_Transfer[22],0,8)BTD(Q5X.Write.BDC[2].Delay_Mode,0,Port_Data.Data_Transfer[23],0,8)MOV(Port,Port_Data.Data_Transfer[185])MOV(0,Port_Data.Data_Transfer[187])MOV(66,Port_Data.Data_Transfer[188])MOV(24,Port_Data.Data_Transfer[189])MOV(11,Inprocess_Index)OTL(Port_Data.Port_Write.[Port])OTL(Local_Control.11);
